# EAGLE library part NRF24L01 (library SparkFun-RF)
Nordic nrf24L01 2.4GHz Low-power Transceiver This is the very popular, low cost, very low power RF transceiver from Nordic Semiconductor. Simple SPI interface. SparkFun Products 2.4GHz Transceiver IC - nRF24L01+ (COM-00690) SparkFun Transceiver Breakout - nRF24L01+ (RP-SMA) (WRL-00705) SparkFun Transceiver Breakout - nRF24L01+ (COM-00691)
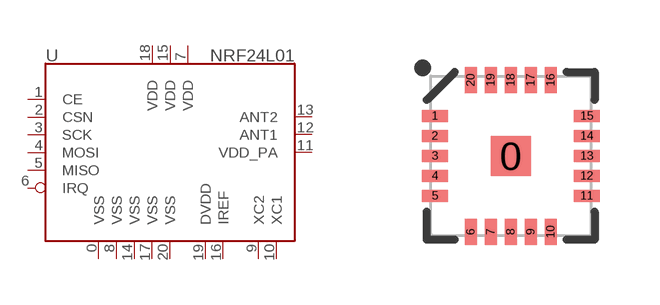
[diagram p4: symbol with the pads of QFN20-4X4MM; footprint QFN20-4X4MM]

Designator prefix -

## NRF24L01SMD (PROD_ID: IC-08950; SF_ID: COM-00690)  [QFN20-4X4MM]
0  VSS  pwr
1  CE  in
2  CSN  in
3  SCK  in
4  MOSI  in
5  MISO  out
6  IRQ  out
7  VDD  pwr
8  VSS  pwr
9  XC2  in
10  XC1  in
11  VDD_PA  pwr
12  ANT1  out
13  ANT2  out
14  VSS  pwr
15  VDD  pwr
16  IREF  in
17  VSS  pwr
18  VDD  pwr
19  DVDD  pwr
20  VSS  pwr

## Footprint QFN20-4X4MM (pad centres in mm)
QFN 20-pin, 4x4mm Used by nRF24L01 Datasheet Example
smd 1 x 1: 0 0,0
smd 0.65 x 0.3: 1 -1.9,1; 2 -1.9,0.5; 3 -1.9,0; 4 -1.9,-0.5; 5 -1.9,-1; 11 1.9,-1; 12 1.9,-0.5; 13 1.9,0; 14 1.9,0.5; 15 1.9,1
smd 0.3 x 0.65: 6 -1,-1.9; 7 -0.5,-1.9; 8 0,-1.9; 9 0.5,-1.9; 10 1,-1.9; 16 1,1.9; 17 0.5,1.9; 18 0,1.9; 19 -0.5,1.9; 20 -1,1.9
